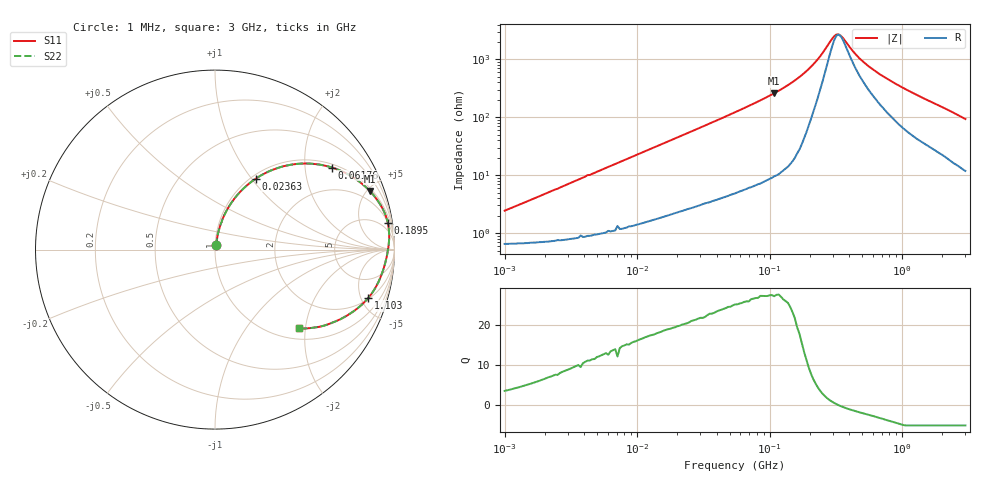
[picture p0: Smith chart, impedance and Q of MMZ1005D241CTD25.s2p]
! S-Parameter Data Generated by TDK Corporation
! Copyright(C) 2025 TDK Corporation.
! All Rights Reserved.
! TDK P/N: MMZ1005D241CTD25 (Chip Bead)
! Property: |Z|=240ohm at 100MHz
! Size(LxWxT): 1x0.5x0.5mm
! Model Type: s2p (Touchstone File Format Version 1.0)
! Frequency: DC=Yes Start=1MHz Stop=3000MHz 202points Log-sweep
! Model Generated on Feb. 6, 2025
! Terms and conditions regarding TDK Simulation Models:
! 1)This simulation model is being provided solely for informational
!  purposes. Please refer to the specifications of the products in
!  terms of detailed characteristics of such products.
! 2)In no event shall TDK Corporation of any of its subsidiaries be
!  liable for any loss or damage arising, directly or indirectly,
!  from any information contained in this simulation model, including,
!  but not limited to loss or damages arising from any inaccuracies,
!  omissions or errors in connection with such information.
! 3)Any and all copyrights on this simulation model are owned by
!  TDK Corporation.  Duplication or redistribution of this simulation
!  model without prior written permission from TDK Corporation
!  is prohibited.
! 4)This simulation model is subject to any modification or change
!  without any prior notice.
! 5)Neither TDK Corporation nor any of its subsidiaries shall make any
!  warranty, express or implied, including but not limited to the
!  correctness, implied warranties of merchantability and fitness for
!  a particular purpose with respect to this simulation models.
! 6)The use of this simulation model shall be deemed to have consented
!  to the terms and conditions hereof.
! Port Assignments:
!  1 ---@@@--- 2
! Applicable Conditions:
!  Temperature = 25 degC
!  DC Bias Current = 0 A
!  Small Signal Operation
# Hz S MA R 50
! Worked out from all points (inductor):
!   201 points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, 1 MHz to 3 GHz, reference 50 ohm
!   read as one part in series: L = 373 nH near 1.041 MHz
!   highest Q = 27.5 at 108.2 MHz (marker M1), where L = 383 nH
!   self-resonance near 334.2 MHz
!   S11 on the Smith chart (normalised r, x): 1 MHz: 1.01, +0.05; 23.63 MHz: 1.05, +1.05; 61.76 MHz: 1.11, +2.77; 189.5 MHz: 2, +13; 1.103 GHz: 2.11, -5.73; 3 GHz: 1.24, -1.85
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1000000  0.02423 73.2  0.9933 -1.3  0.9933 -1.3  0.02423 73.2
3900413  0.08947 79.5  0.9876 -5.1  0.9876 -5.1  0.08947 79.5
7110411  0.158 76.3  0.9746 -9.1  0.9746 -9.1  0.158 76.3
1.461624e7  0.3069 69.0  0.935 -17.8  0.935 -17.8  0.3069 69.0
2.362996e7  0.4559 60.1  0.8681 -27.1  0.8681 -27.1  0.4559 60.1
3.670325e7  0.6176 49.4  0.76 -38.1  0.76 -38.1  0.6176 49.4
5.477226e7  0.7589 38.4  0.6218 -49.3  0.6218 -49.3  0.7589 38.4
6.176144e7  0.7959 35.1  0.5751 -52.7  0.5751 -52.7  0.7959 35.1
1.081723e8  0.9223 20.7  0.3542 -67.2  0.3542 -67.2  0.9223 20.7
1.49005e8  0.9615 13.7  0.2365 -73.9  0.2365 -73.9  0.9615 13.7
1.894586e8  0.9743 8.9  0.1552 -76.1  0.1552 -76.1  0.9743 8.9
2.136344e8  0.9752 6.7  0.1185 -74.6  0.1185 -74.6  0.9752 6.7
2.408952e8  0.9738 4.7  0.08563 -69.8  0.08563 -69.8  0.9738 4.7
3.062963e8  0.9671 1.2  0.03857 -30.9  0.03857 -30.9  0.9671 1.2
3.318279e8  0.9643 0.1  0.03576 -2.3  0.03576 -2.3  0.9643 0.1
3.594878e8  0.9616 -0.9  0.04167 22.4  0.04167 22.4  0.9616 -0.9
4.391493e8  0.9543 -3.5  0.07506 50.8  0.07506 50.8  0.9543 -3.5
4.951867e8  0.9497 -5.0  0.09891 57.0  0.09891 57.0  0.9497 -5.0
8.005644e8  0.9258 -11.8  0.2113 63.7  0.2113 63.7  0.9258 -11.8
1.10276e9  0.8952 -17.5  0.3068 61.5  0.3068 61.5  0.8952 -17.5
1.855641e9  0.7997 -29.0  0.4903 52.2  0.4903 52.2  0.7997 -29.0
3e9  0.6429 -43.1  0.6888 39.6  0.6888 39.6  0.6429 -43.1
